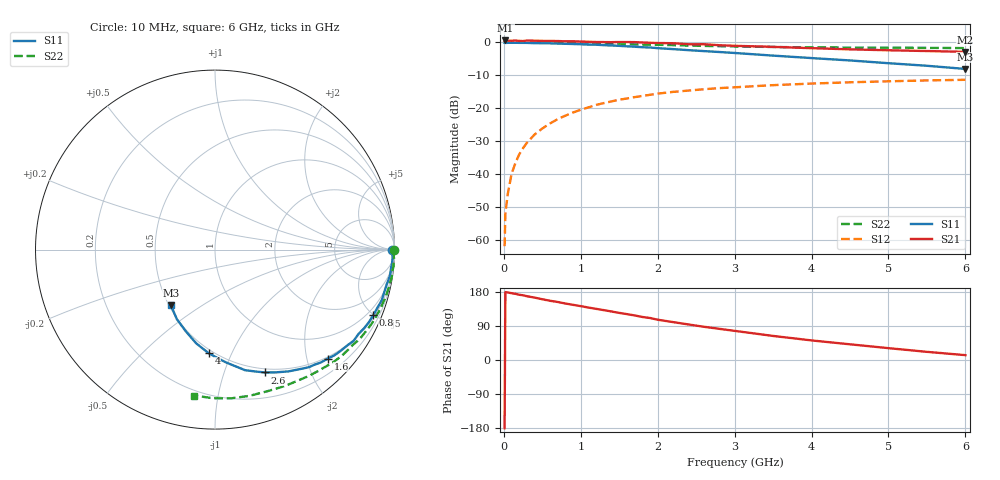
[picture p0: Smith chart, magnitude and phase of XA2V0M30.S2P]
! SIEMENS Discrete & RF Semiconductors
! BFY180
! Si NPN RF Bipolar Junction Transistor in MICRO-X
! VCE = 2 V  IC = 0.3 mA
! Common Emitter S-Parameters:  May  1997
# GHz  S  MA  R  50
!  f  S11  S21  S12  S22
! GHz  MAG  ANG  MAG  ANG  MAG  ANG  MAG  ANG
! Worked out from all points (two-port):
!   36 points, 10 MHz to 6 GHz, reference 50 ohm
!   highest |S21| = 0.61 dB at 20 MHz (marker M1); lowest = -2.9 dB at 6 GHz (marker M2)
!   |S21| within 3 dB of the highest: start of sweep to 5.034 GHz
!   lowest |S11| = -8.1 dB at 6 GHz (marker M3), VSWR 2.31, Z = 25.6 - j18.8 ohm
!   |S11| at or under -10 dB: nowhere
!   |S22| runs from -1.7 to 0.0 dB; largest |S21 - S12| = 1.1
!   S11 on the Smith chart (normalised r, x): 10 MHz: open; 800 MHz: 0.60, -4.96; 1.6 GHz: 0.47, -2.40; 2.6 GHz: 0.46, -1.39; 4 GHz: 0.47, -0.82; 6 GHz: 0.51, -0.38
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0.01  0.9877 -0.1  1.047 -180.0  0.0008 86.8  0.9998 -0.2
0.02  0.9837 -0.7  1.073 179.2  0.0025 93.0  0.9999 -0.4
0.05  0.9873 -1.3  1.064 178.3  0.0049 87.9  0.9992 -1.0
0.1  0.9904 -2.6  1.062 176.3  0.01 92.9  0.9965 -2.1
0.15  0.9897 -4.3  1.069 174.6  0.0147 87.2  0.9999 -3.2
0.2  0.9864 -5.6  1.058 172.2  0.0199 85.7  0.998 -4.2
0.25  0.9862 -7.2  1.051 170.8  0.0248 84.2  0.9997 -5.4
0.3  0.9855 -8.5  1.069 168.3  0.0298 82.9  0.9961 -6.4
0.4  0.9762 -11.4  1.064 164.7  0.0399 80.8  0.9965 -8.4
0.5  0.9725 -14.2  1.057 160.3  0.0492 78.7  0.9933 -10.6
0.8  0.9544 -22.5  1.041 149.1  0.0771 71.4  0.9839 -16.8
1.1  0.9274 -30.4  1.025 138.4  0.1031 64.5  0.9703 -22.9
1.6  0.8737 -44.0  1.014 121.1  0.1408 53.7  0.9423 -32.8
1.8  0.8469 -49.3  1 113.6  0.1539 49.8  0.9296 -36.4
2.2  0.7925 -58.9  0.974 100.0  0.1773 42.1  0.9102 -43.5
2.6  0.7394 -67.8  0.941 87.7  0.1943 35.7  0.8867 -49.9
3  0.6924 -76.0  0.89 76.9  0.2082 29.5  0.8685 -55.9
3.5  0.6312 -84.5  0.857 63.5  0.2244 23.1  0.8541 -62.8
4  0.5791 -93.4  0.819 51.7  0.2372 16.9  0.8413 -69.7
4.5  0.5329 -101.3  0.786 41.4  0.2481 11.4  0.8372 -76.7
5.5  0.4423 -118.7  0.741 21.5  0.2648 0.6  0.8282 -90.9
6  0.3958 -128.4  0.72 12.8  0.2707 -4.8  0.821 -98.0
